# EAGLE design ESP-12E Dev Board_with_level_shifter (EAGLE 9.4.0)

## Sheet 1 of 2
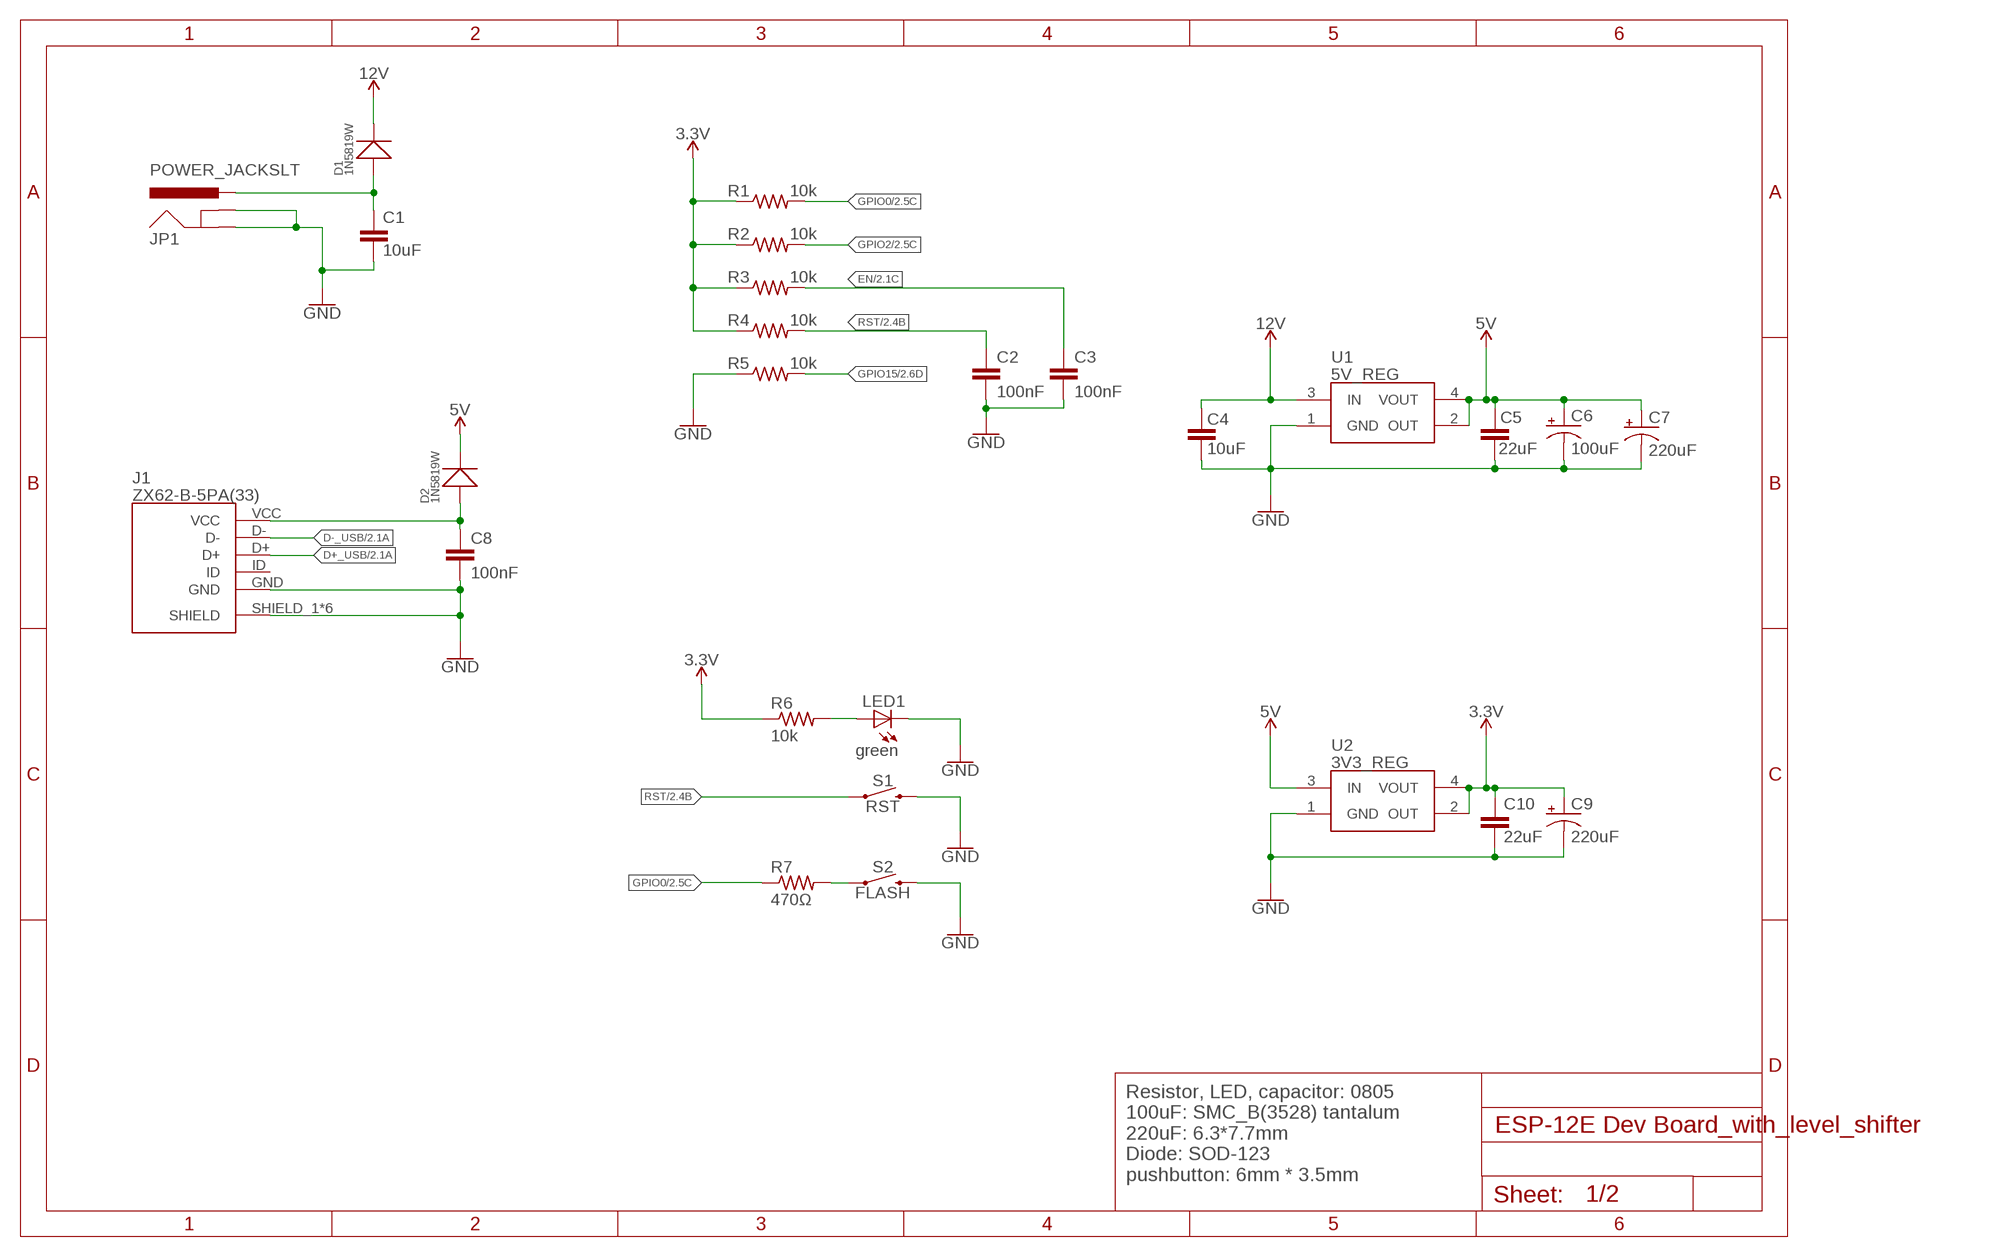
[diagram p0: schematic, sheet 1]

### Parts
C1  10uF  C-EUC0805  [C0805]
C2  100nF  C-EUC0805  [C0805]
C3  100nF  C-EUC0805  [C0805]
C4  10uF  C-EUC0805  [C0805]
C5  22uF  C-EUC0805  [C0805]
C6  100uF  CPOL-USSMCB  [SMC_B]
C7  220uF  CPOL-USUD-6,3X7,7  [UD-6,3X7,7_NICHICON]
C8  100nF  C-EUC0805  [C0805]
C9  220uF  CPOL-USUD-6,3X7,7  [UD-6,3X7,7_NICHICON]
C10  22uF  C-EUC0805  [C0805]
D1  1N5819W  SMD-DIODE-SCHOTTKY-20V-500MA(SOD-123)  [SOD-123]
D2  1N5819W  SMD-DIODE-SCHOTTKY-20V-500MA(SOD-123)  [SOD-123]
J1  ZX62-B-5PA(33)  [ZX62B5PA33]
JP1  POWER_JACKSLT  [POWER_JACK_SLOT]
LED1  green  LEDCHIP-LED0805  [CHIP-LED0805]
R1  10k  R-US_R0805  [R0805]
R2  10k  R-US_R0805  [R0805]
R3  10k  R-US_R0805  [R0805]
R4  10k  R-US_R0805  [R0805]
R5  10k  R-US_R0805  [R0805]
R6  10k  R-US_R0805  [R0805]
R7  470Ω  R-US_R0805  [R0805]
S1  RST  MOMENTARY-SWITCH-SPST-SMD-6.0X3.5MM  [TACTILE_SWITCH_SMD_6.0X3.5MM]
S2  FLASH  MOMENTARY-SWITCH-SPST-SMD-6.0X3.5MM  [TACTILE_SWITCH_SMD_6.0X3.5MM]
U1  5V_REG  AZ1117H-5.0TRE1  [SOT230P700X170-4N]
U2  3V3_REG  AZ1117H-5.0TRE1  [SOT230P700X170-4N]

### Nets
3.3V [power]: C9.+ C10.2 R1.1 R2.1 R3.1 R4.1 R6.1 U2.2(OUT) U2.4(VOUT) ; also sheet 2
5V [power]: C5.1 C6.+ C7.+ D2.- U1.2(OUT) U1.4(VOUT) U2.3(IN) ; also sheet 2
12V [power]: C4.1 D1.- U1.3(IN) ; also sheet 2
D+_USB: J1.D+ ; also sheet 2
D-_USB: J1.D- ; also sheet 2
EN: C3.2 R3.2 ; also sheet 2
GND [power]: C1.1 C2.1 C3.1 C4.2 C5.2 C6.- C7.- C8.1 C9.- C10.1 J1.GND J1.SHIELD_1(SHIELD) J1.SHIELD_2(SHIELD) J1.SHIELD_3(SHIELD) J1.SHIELD_4(SHIELD) J1.SHIELD_5(SHIELD) J1.SHIELD_6(SHIELD) JP1.GND@1(GNDBREAK) JP1.GND@2(GND) LED1.C R5.1 S1.2 S2.2 U1.1(GND) U2.1(GND) ; also sheet 2
GPIO0: R1.2 R7.1 ; also sheet 2
GPIO2: R2.2 ; also sheet 2
GPIO15: R5.2 ; also sheet 2
N$3: C1.2 D1.+ JP1.PWR
N$4: LED1.A R6.2
N$10 [power]: C8.2 D2.+ J1.VCC
POWER1: R7.2 S2.1
RST: C2.2 R4.2 S1.1 ; also sheet 2
Unconnected: J1.ID

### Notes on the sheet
- Resistor, LED, capacitor: 0805
  100uF: SMC_B(3528) tantalum
  220uF: 6.3*7.7mm
  Diode: SOD-123
  pushbutton: 6mm * 3.5mm

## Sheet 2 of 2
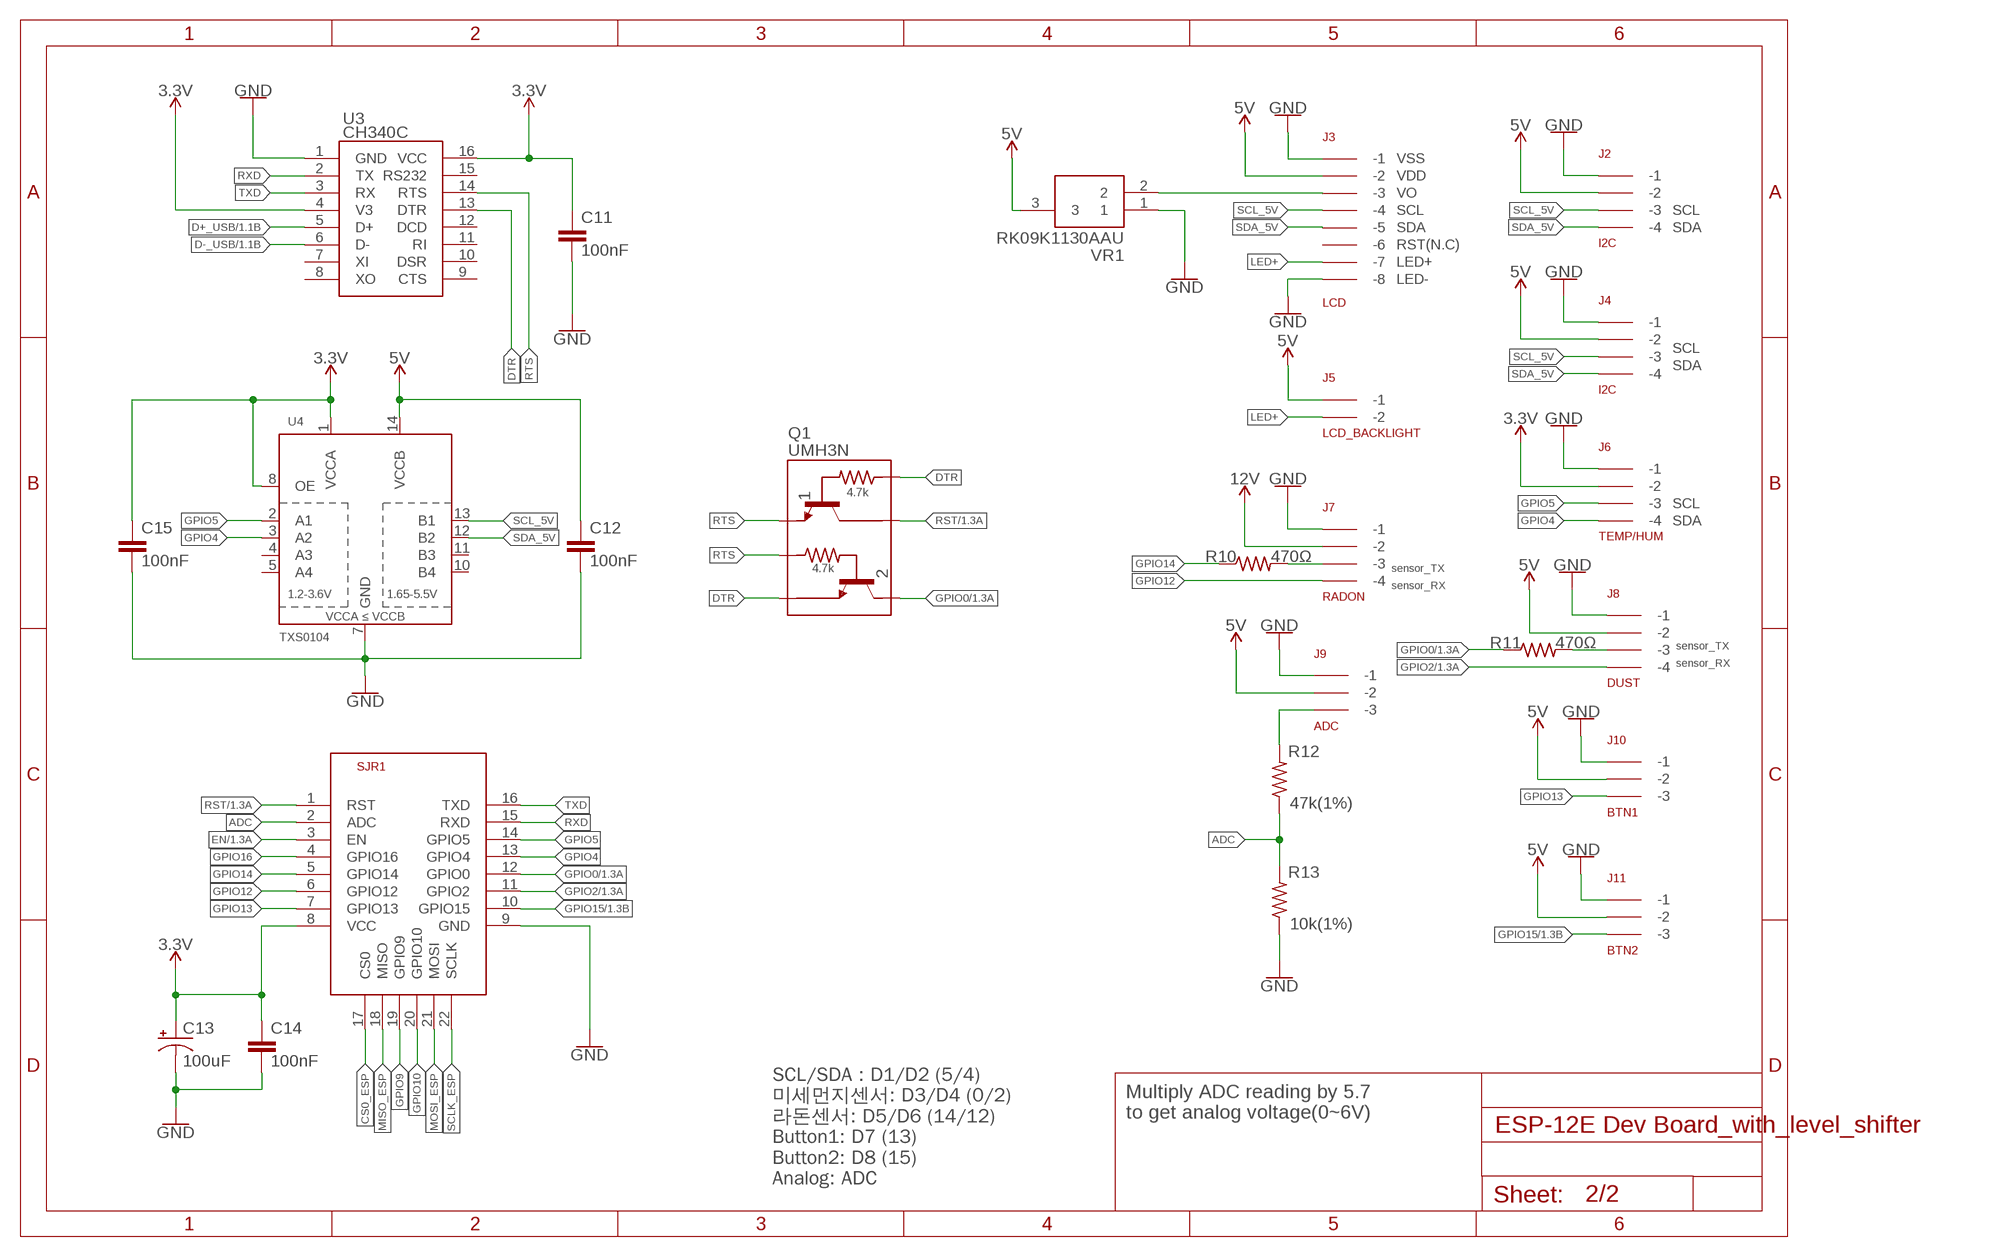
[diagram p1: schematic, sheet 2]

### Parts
C11  100nF  C-EUC0805  [C0805]
C12  100nF  C-EUC0805  [C0805]
C13  100uF  CPOL-USSMCB  [SMC_B]
C14  100nF  C-EUC0805  [C0805]
C15  100nF  C-EUC0805  [C0805]
J2  I2C  5267-4  [5267-4]
J3  LCD  5267-8  [5267-8]
J4  I2C  5267-4  [5267-4]
J5  LCD_BACKLIGHT  5267-2  [5267-2]
J6  TEMP/HUM  5267-4  [5267-4]
J7  RADON  5267-4  [5267-4]
J8  DUST  5267-4  [5267-4]
J9  ADC  5267-3  [5267-3]
J10  BTN1  5267-3  [5267-3]
J11  BTN2  5267-3  [5267-3]
Q1  UMH3N  UMH3NFHATN  [SOT65P210X100-6N]
R10  470Ω  R-US_R0805  [R0805]
R11  470Ω  R-US_R0805  [R0805]
R12  47k(1%)  R-US_R0805  [R0805]
R13  10k(1%)  R-US_R0805  [R0805]
SJR1  ESP-12E  ESP8266-12EESP12E  [ESP8266-ESP12E]
U3  CH340C  CH340G  [SOIC16]
U4  TXS0104  TXB0104PWR  [TSSOP14]
VR1  RK09K1130AAU  RK09K1130A6S  [RK09K1130BGM]

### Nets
3.3V [power]: C11.2 C13.+ C14.2 C15.2 J6.P$2(-2) SJR1.8(VCC) U3.4(V3) U3.16(VCC) U4.1(VCCA) U4.8(OE) ; also sheet 1
5V [power]: C12.2 J2.P$2(-2) J3.P$2(-2) J4.P$2(-2) J5.P$1(-1) J8.P$2(-2) J9.P$2(-2) J10.P$2(-2) J11.P$2(-2) U4.14(VCCB) VR1.3 ; also sheet 1
12V [power]: J7.P$2(-2) ; also sheet 1
ADC: R12.1 R13.2 SJR1.2(ADC)
CS0_ESP: SJR1.17(CS0)
D+_USB: U3.5(D+) ; also sheet 1
D-_USB: U3.6(D-) ; also sheet 1
DTR: Q1.2 Q1.4 U3.13(DTR)
EN: SJR1.3(EN) ; also sheet 1
GND [power]: C11.1 C12.1 C13.- C14.1 C15.1 J2.P$1(-1) J3.P$1(-1) J3.P$8(-8) J4.P$1(-1) J6.P$1(-1) J7.P$1(-1) J8.P$1(-1) J9.P$1(-1) J10.P$1(-1) J11.P$1(-1) R13.1 SJR1.9(GND) U3.1(GND) U4.7(GND) VR1.1 ; also sheet 1
GPIO0: Q1.3 R11.1 SJR1.12(GPIO0) ; also sheet 1
GPIO2: J8.P$4(-4) SJR1.11(GPIO2) ; also sheet 1
GPIO4: J6.P$4(-4) SJR1.13(GPIO4) U4.3(A2)
GPIO5: J6.P$3(-3) SJR1.14(GPIO5) U4.2(A1)
GPIO9: SJR1.19(GPIO9)
GPIO10: SJR1.20(GPIO10)
GPIO12: J7.P$4(-4) SJR1.6(GPIO12)
GPIO13: J10.P$3(-3) SJR1.7(GPIO13)
GPIO14: R10.1 SJR1.5(GPIO14)
GPIO15: J11.P$3(-3) SJR1.10(GPIO15) ; also sheet 1
GPIO16: SJR1.4(GPIO16)
LED+: J3.P$7(-7) J5.P$2(-2)
MISO_ESP: SJR1.18(MISO)
MOSI_ESP: SJR1.21(MOSI)
N$2: J3.P$3(-3) VR1.2
N$5: J9.P$3(-3) R12.2
N$6: J7.P$3(-3) R10.2
N$9: J8.P$3(-3) R11.2
RST: Q1.6 SJR1.1(RST) ; also sheet 1
RTS: Q1.1 Q1.5 U3.14(RTS)
RXD: SJR1.15(RXD) U3.2(TX)
SCL_5V: J2.P$3(-3) J3.P$4(-4) J4.P$3(-3) U4.13(B1)
SCLK_ESP: SJR1.22(SCLK)
SDA_5V: J2.P$4(-4) J3.P$5(-5) J4.P$4(-4) U4.12(B2)
TXD: SJR1.16(TXD) U3.3(RX)
Unconnected: J3.P$6(-6) U3.7(XI) U3.8(XO) U3.9(CTS) U3.10(DSR) U3.11(RI) U3.12(DCD) U3.15(RS232) U4.4(A3) U4.5(A4) U4.10(B4) U4.11(B3)

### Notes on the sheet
- VSS
- VDD
- VO
- SCL | SCL
- SDA | SDA
- RST(N.C)
- LED+
- LED-
- SCL
- SDA
- SCL
- SDA
- sensor_TX
- sensor_RX
- sensor_TX
- sensor_RX
- SCL/SDA : D1/D2 (5/4)
  미세먼지센서: D3/D4 (0/2)
  라돈센서: D5/D6 (14/12)
  Button1: D7 (13)
  Button2: D8 (15)
  Analog: ADC
- Multiply ADC reading by 5.7
  to get analog voltage(0~6V)

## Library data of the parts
C1-C5 C8 C10-C12 C14 C15 = rcl:C-EU: CAPACITOR, European symbol; SPICEPREFIX: C
C6 C7 C9 C13 = rcl:CPOL-US: POLARIZED CAPACITOR, American symbol; SPICEPREFIX: C
D1 D2 = Seeed-Diode:SMD-DIODE-SCHOTTKY-20V-500MA(SOD-123): 304020032; MPN: SS0520-7-F; VALUE: 20V-500MA
J1 = SamacSys_Parts:ZX62-B-5PA(33): USB Connectors MICRO B RECEPT RA SMT BTTM MNT Source: Datasheet; DESCRIPTION: USB Connectors MICRO B RECEPT RA SMT BTTM MNT; HEIGHT: 2.8mm; MANUFACTURER_NAME: Hirose; MANUFACTURER_PART_NUMBER: ZX62-B-5PA(33); MOUSER_PART_NUMBER: 798-ZX62-B-5PA33; MOUSER_PRICE-STOCK: https://www.mouser.com/Search/Refine.aspx?Keyword=798-ZX62-B-5PA33
J2 J4 J6-J8 = con-molex-spox:5267-4
J3 = con-molex-spox:5267-8
J5 = con-molex-spox:5267-2
J9-J11 = con-molex-spox:5267-3
JP1 = kanflo:POWER_JACK: Power Jack This is the standard 5.5mm barrel jack for power. The SLT footprint has been proven in designs produced by DirtyPCBs.com and only works if the mill layer is transmitted to the PCB fab house and the fab house accepts it. Rumours has it OSH Park accepts this design too. This symbol is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
LED1 = adafruit:LED: LED
Q1 = SamacSys_Parts:UMH3NFHATN: ROHM - UMH3NFHATN - TRANS, NPN, AUTO, 4.7K/4.7K, SOT-353 Source: Datasheet; DESCRIPTION: ROHM - UMH3NFHATN - TRANS, NPN, AUTO, 4.7K/4.7K, SOT-353; HEIGHT: 1mm; MANUFACTURER_NAME: ROHM Semiconductor; MANUFACTURER_PART_NUMBER: UMH3NFHATN; MOUSER_PART_NUMBER: 755-UMH3NFHATN; MOUSER_PRICE-STOCK: https://www.mouser.com/Search/Refine.aspx?Keyword=755-UMH3NFHATN
R1-R7 R10-R13 = rcl:R-US_: RESISTOR, American symbol; SPICEPREFIX: R
S1 S2 = SparkFun-Switches:MOMENTARY-SWITCH-SPST: Momentary Switch (Pushbutton) - SPST; PROD_ID: SWCH-00815; SF_SKU: COM-08229
SJR1 = esp12e:ESP8266-12E: ESP8266-12E Library for Eagle CAD The author not responsible for any damages or errors!. Created by Suhail jr.lt;/author>
U1 U2 = SamacSys_Parts:AZ1117H-5.0TRE1: 1A 5V LDO Linear Voltage Reg SOT-223 Diodes Inc AZ1117H-5.0TRE1, Single Linear Voltage Regulator, 1A 4.9 5.1 V, 1%, 3-Pin SOT-223 Source: Datasheet; DESCRIPTION: 1A 5V LDO Linear Voltage Reg SOT-223 Diodes Inc AZ1117H-5.0TRE1, Single Linear Voltage Regulator, 1A 4.9 5.1 V, 1%, 3-Pin SOT-223; HEIGHT: 1.7mm; MANUFACTURER_NAME: Diodes Inc.; MANUFACTURER_PART_NUMBER: AZ1117H-5.0TRE1; MOUSER_PART_NUMBER: 621-AZ1117H-5.0TRE1; MOUSER_PRICE-STOCK: https://www.mouser.com/Search/Refine.aspx?Keyword=621-AZ1117H-5.0TRE1
U3 = ch340g:CH340G
U4 = SparkFun-IC-Comms:TXB0104PWR: 4-Bit Bi-Directional Level Shifter 1.2V-3.6V (VCCA) to 1.65V-5.5V (VCCB) bi-directional level shifter with auto direction sensing. Max data rate - VCCA 1.8V: 20Mbps (50ns), VCCA 3.3V: 100Mbps (10ns) Digikey: 296-21929-1-ND (TSSOP) Datasheet SparkFun Products SparkFun Cellular Shield - MG2639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; PROD_ID: NA-XXXXX; VALUE: TXB0104
VR1 = SamacSys_Parts:RK09K1130A6S: Audio single pot. 10K Vertical 15mm,1B Alps RK09K Series, Linear Potentiometer with a 6 mm Dia. Shaft, 10k, +/-20%, Through Hole Source: Datasheet; DESCRIPTION: Audio single pot. 10K Vertical 15mm,1B Alps RK09K Series, Linear Potentiometer with a 6 mm Dia. Shaft, 10k, +/-20%, Through Hole; HEIGHT: mm; MANUFACTURER_NAME: ALPS; MANUFACTURER_PART_NUMBER: RK09K1130A6S; MOUSER_PART_NUMBER: 688-RK09K1130A6S; MOUSER_PRICE-STOCK: https://www.mouser.com/Search/Refine.aspx?Keyword=688-RK09K1130A6S

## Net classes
1 power: width 0.457 mm

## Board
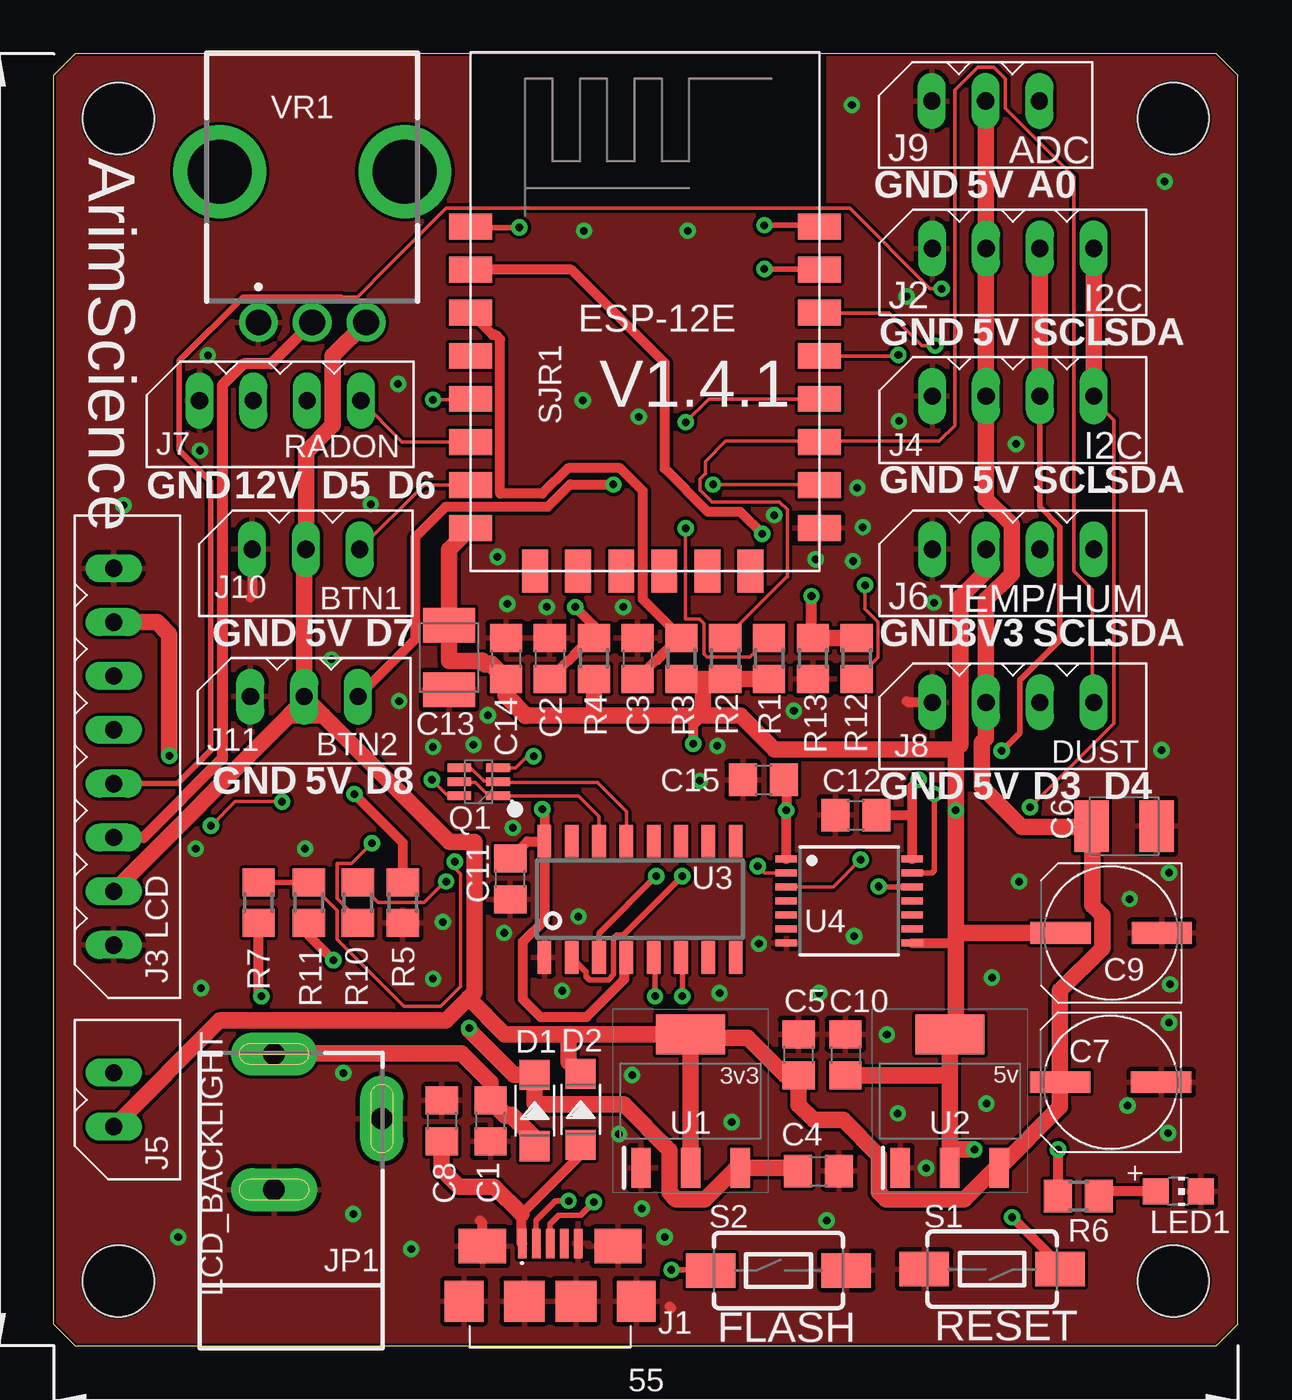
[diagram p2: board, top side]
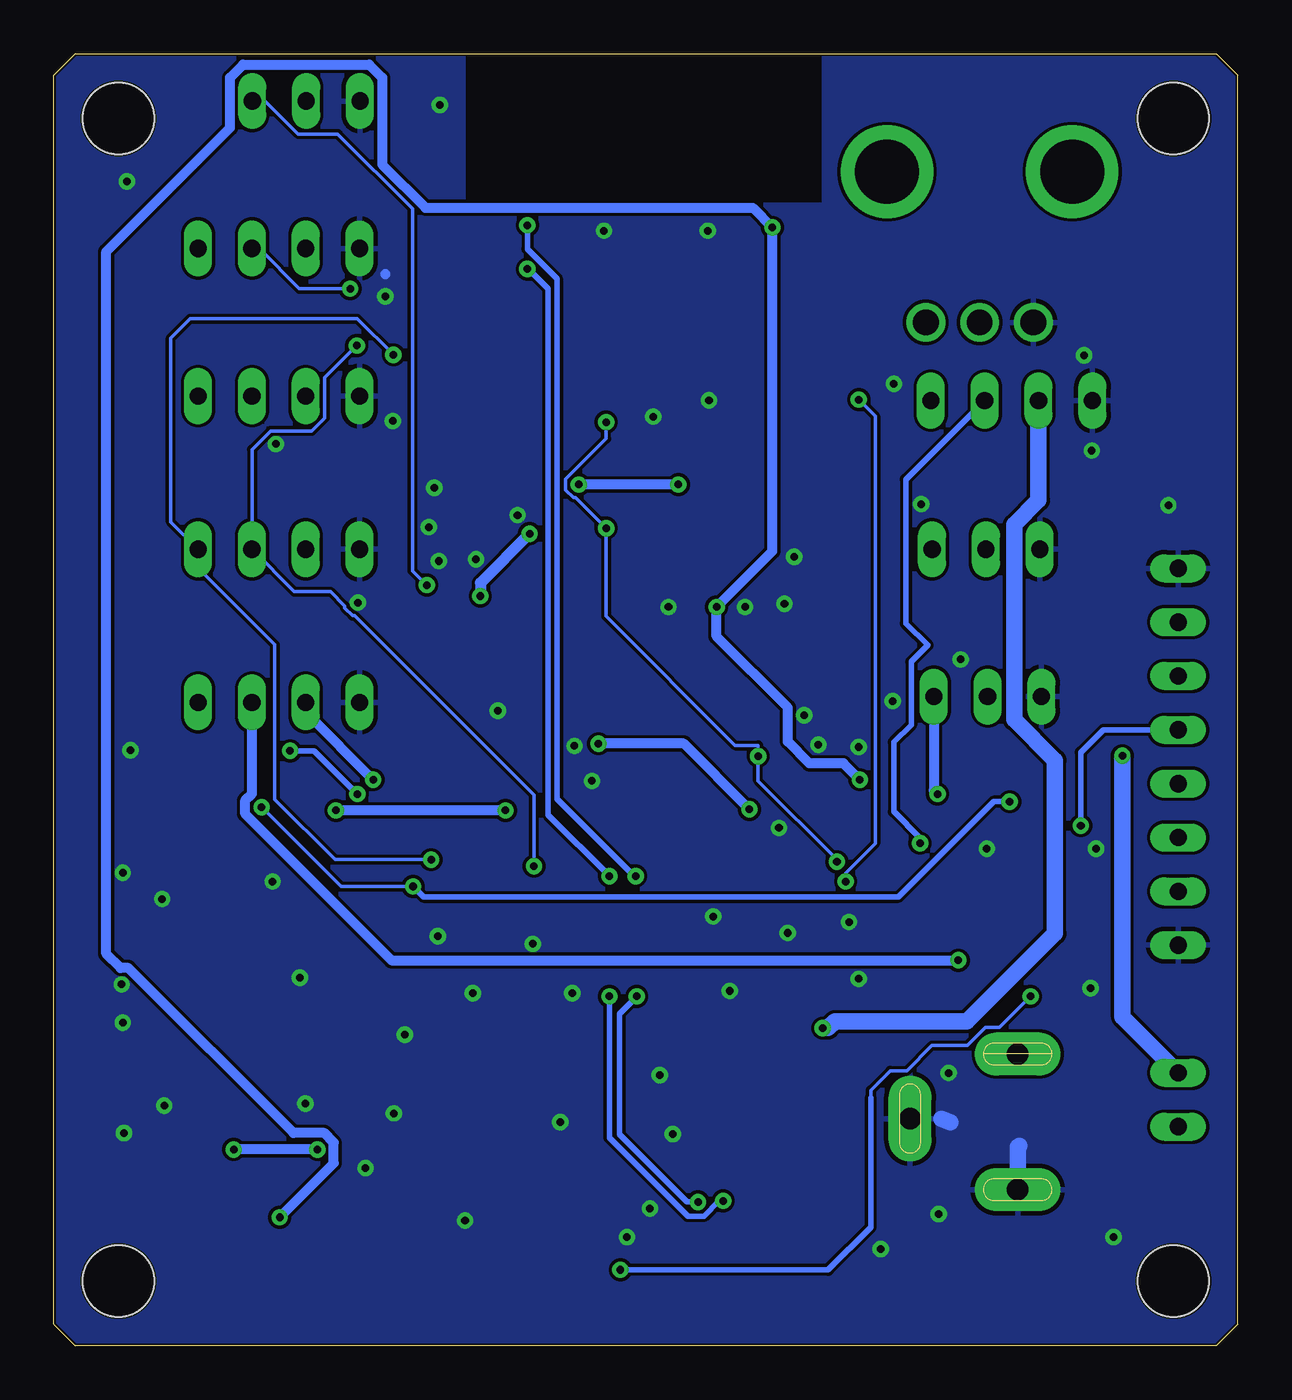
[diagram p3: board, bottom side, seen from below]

Size 55 x 60 mm. Coordinates in mm from the lower left corner, seen from the top.
Outline: 0,1 0,59 1,60 54,60 55,59 55,1 54,0 1,0 0,1
Copper layers (1*16): Top 0.035mm / dielectric 1.5mm / Bottom 0.035mm
Design rules "default *": minimum track width 6mil, minimum drill 0.35mm, track to track 6mil, track to pad 6mil, pad to pad 6mil, via to via 6mil, smd to smd 6mil, copper to edge 4mil, drill to drill 6mil, minimum pad ring 10mil, minimum via ring 8mil, stop-mask expansion 4mil, vias tented up to drill 15mil, thermal gap 8mil
Holes 3.3 mm at 3,57 52,57 52,3 3,3

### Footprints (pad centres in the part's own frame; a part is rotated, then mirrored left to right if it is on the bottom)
C0805 = smd 1.3 x 1.5: 1 -0.95,0; 2 0.95,0
SMC_B = smd 1.6 x 2.4: + -1.5,0; - 1.5,0
UD-6,3X7,7_NICHICON = smd 2.8 x 1: + 2.35,0; - -2.35,0
SOD-123 = smd 1.397 x 1.397: + -1.651,0; - 1.651,0
ZX62B5PA33 = smd 0.4 x 1.35: D+ 0,1.95; D- -0.65,1.95; GND 1.3,1.95; ID 0.65,1.95; VCC -1.3,1.95 | smd 2.2 x 1.6: SHIELD_1 -3.15,1.825; SHIELD_6 3.15,1.825 | smd 1.8 x 1.9: SHIELD_2 -4,-0.725; SHIELD_5 4,-0.725 | smd 1.9 x 1.9: SHIELD_3 -1.2,-0.725; SHIELD_4 1.2,-0.725
5267-4 = drill 0.8 long: P$1 0,0; P$2 2.5,0; P$3 5,0; P$4 7.5,0
5267-8 = drill 0.8 long: P$1 0,0; P$2 2.5,0; P$3 5,0; P$4 7.5,0; P$5 10,0; P$6 12.5,0; P$7 15,0; P$8 17.5,0
5267-2 = drill 0.8 long: P$1 0,0; P$2 2.5,0
5267-3 = drill 0.8 long: P$1 0,0; P$2 2.5,0; P$3 5,0
POWER_JACK_SLOT = drill 1 pad 2 long: GND@1 2.5,1.39; GND@2 -2.5,-1.91; PWR 2.5,-4.91
CHIP-LED0805 = smd 1.2 x 1.2: A 0,-1.05; C 0,1.05
SOT65P210X100-6N = smd 1.1 x 0.4: 1 -0.9,0.65; 2 -0.9,0; 3 -0.9,-0.65; 4 0.9,-0.65; 5 0.9,0; 6 0.9,0.65
R0805 = smd 1.3 x 1.5: 1 -0.95,0; 2 0.95,0
TACTILE_SWITCH_SMD_6.0X3.5MM = smd 2.3 x 1.6: 1 -3.15,0; 2 3.15,0
ESP8266-ESP12E = smd 2 x 1.2: 1 -7.62,5.84; 2 -7.62,3.84; 3 -7.62,1.84; 4 -7.62,-0.16; 5 -7.62,-2.16; 6 -7.62,-4.16; 7 -7.62,-6.16; 8 -7.62,-8.16; 9 8.58,-8.16; 10 8.58,-6.16; 11 8.58,-4.16; 12 8.58,-2.16; 13 8.58,-0.16; 14 8.58,1.84; 15 8.58,3.84; 16 8.58,5.84 | smd 1.2 x 2: 17 -4.62,-10.16; 18 -2.62,-10.16; 19 -0.62,-10.16; 20 1.38,-10.16; 21 3.38,-10.16; 22 5.38,-10.16
SOT230P700X170-4N = smd 1.85 x 0.9: 1 -3.1,2.3; 2 -3.1,0; 3 -3.1,-2.3 | smd 1.85 x 3.2: 4 3.1,0
SOIC16 = smd 0.635 x 1.524: 1 -4.445,-2.695; 2 -3.175,-2.695; 3 -1.905,-2.695; 4 -0.635,-2.695; 5 0.635,-2.695; 6 1.905,-2.695; 7 3.175,-2.695; 8 4.445,-2.695; 9 4.445,2.695; 10 3.175,2.695; 11 1.905,2.695; 12 0.635,2.695; 13 -0.635,2.695; 14 -1.905,2.695; 15 -3.175,2.695; 16 -4.445,2.695
TSSOP14 = smd 0.305 x 0.991: 1 -1.95,-2.918; 2 -1.3,-2.918; 3 -0.65,-2.918; 4 0,-2.918; 5 0.65,-2.918; 6 1.3,-2.918; 7 1.95,-2.918; 8 1.95,2.918; 9 1.3,2.918; 10 0.65,2.918; 11 0,2.918; 12 -0.65,2.918; 13 -1.3,2.918; 14 -1.95,2.918
RK09K1130BGM = drill 1.2 pad 1.8: 1 -2.5,-12.5; 2 0,-12.5; 3 2.5,-12.5 | drill 2.97 pad 4.3: 4 4.3,-5.5; 5 -4.3,-5.5

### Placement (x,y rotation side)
C1  20.29,10.43 90 top
C2  23.03,31.92 270 top
C3  27.11,31.92 270 top
C4  35.52,8.11 0 top
C5  34.59,13.51 90 top
C6  49.71,24.13 0 top
C7  49.08,12.23 180 top
C8  18.02,10.43 270 top
C9  49.11,19.17 180 top
C10  36.77,13.51 270 top
C11  21.2,21.68 90 top
C12  37.24,24.64 0 top
C13  18.36,31.96 270 top
C14  21,31.91 270 top
C15  32.95,26.28 0 top
D1  22.34,10.92 90 top
D2  24.47,10.97 90 top
J1  23.05,2.79 0 top
J2  40.8,50.96 0 top
J3  2.78,18.6 90 top
J4  40.8,44.1 0 top
J5  2.78,10.17 90 top
J6  40.8,36.99 0 top
J7  6.76,43.9 0 top
J8  40.8,29.88 0 top
J9  40.78,57.81 0 top
J10  9.21,36.99 0 top
J11  9.13,30.15 0 top
JP1  12.73,8.64 180 top
LED1  52.23,7.16 270 top
Q1  19.73,26.19 180 top
R1  33.22,31.92 90 top
R2  31.19,31.92 90 top
R3  29.15,31.92 90 top
R4  25.09,31.92 90 top
R5  16.21,20.57 90 top
R6  47.59,6.95 0 top
R7  9.51,20.57 270 top
R10  14.13,20.57 270 top
R11  11.84,20.57 270 top
R12  37.29,31.92 270 top
R13  35.26,31.92 90 top
S1  43.58,3.56 180 top
S2  33.65,3.49 0 top
SJR1  26.97,46.13 0 top
U1  29.57,11.37 90 top
U2  41.61,11.37 90 top
U3  27.23,20.73 0 top
U4  36.94,20.66 270 top
VR1  12,60.02 0 top

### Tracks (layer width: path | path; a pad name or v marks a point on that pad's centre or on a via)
3.3V  (via drill 0.35)
  Top 0.457: U4.1 v34.02,24.86 | v34.02,24.86 | U4.8 41.85,18.7 41.89,18.66 | v29.7,27.96 29.7,28.82 30.16,29.28 | C11.2 22,23.43 U3.16 | v22.69,24.91 22.78,24.82 U3.16 | U3.4 26.5,17.95 26.5,17.03 24.75,15.27 22.61,15.27 21.78,16.1 21.78,18.76 22.78,19.76 U3.16 | C15.2 34.02,26.16 v34.02,24.86 | v46.64,9.11 R6.1
  Top 0.762: R3.1 30.16,30.97 | 30.16,30.97 R2.1 R1.1 | J6.P$2 43.3,35.95 42.11,34.76 42.11,27.91 41.89,27.69 | v42.76,9.11 41.61,9.11 U2.2 41.61,12.62 | 41.89,27.69 v41.89,24.86 41.89,19.17 | SJR1.8 18.36,36.98 C13.+ 18.36,31.8 18.37,31.79 19.86,31.79 | 30.16,29.28 31.89,29.28 33.48,27.69 41.89,27.69 | 30.16,30.97 30.16,29.28 | 41.89,19.17 41.89,18.66 41.89,14.75 U2.4 41.61,12.62 | C9.+ 41.89,19.17 | C10.2 41.56,12.56 41.61,12.62 | 30.16,29.28 25.08,29.28 | 25.08,29.28 21.92,29.28 | 25.08,29.28 R4.1
  Top 0.813: 21.92,29.28 21,30.2 C14.2 20.31,31.65 20.02,31.65 19.88,31.79 19.86,31.79
  Bottom 0.457: v34.02,24.86 v41.89,24.86 | v22.69,24.91 25.74,27.96 v29.7,27.96 | v42.76,9.11 v46.64,9.11
5V  (via drill 0.35)
  Top 0.457: 39.86,24.66 39.86,25.98 v40.17,26.28 | 39.86,24.66 39.86,22.65 U4.14 | C12.2 38.21,24.66 39.86,24.66
  Top 0.762: J9.P$2 43.28,50.98 J2.P$2 J4.P$2 43.3,39.32 44.49,38.14 44.49,35.84 43.3,34.66 J8.P$2 43.3,28.19 43.12,28.01 43.12,25.96 44.97,24.1 48.18,24.1 C6.+ 48.24,24.09 48.24,20.44 48.69,19.99 48.69,18.45 46.73,16.49 C7.+ 46.73,11.09 U2.3 43.74,8.27 42.28,6.81 38.64,6.81 38.33,7.12 38.33,8.82 36.67,10.48 35.3,10.48 34.59,11.2 C5.1 33.98,12.56 32.24,14.3 29.74,14.3 U1.4 | J11.P$2 11.63,36.91 J10.P$2 11.71,41.51 12.95,42.75 12.95,45.98 VR1.3 | J3.P$2 10.94,29.26 | 10.94,29.26 11.63,29.95 J11.P$2 | J11.P$2 12.51,29.26 | 12.51,29.26 18.38,23.4 19.54,23.4 19.54,16.42 19.27,16.14 | 12.51,29.26 10.94,29.26 | 19.27,16.14 18.23,15.11 7.71,15.11 J5.P$1 | 19.27,16.14 20.94,14.47 23.91,14.47 | U1.4 23.91,14.47 | U1.2 U1.4 | D2.- 23.91,13.18 23.91,14.47
  Bottom 0.457: v40.17,26.28 43.29,29.41 43.29,29.81 J8.P$2
12V  (via drill 0.35)
  Top 0.762: v19.29,14.75 19.29,14.66 21.37,12.57 D1.- 22.34,11.25 22.38,11.2 26.47,11.2 28.59,9.08 28.59,7.12 28.9,6.81 30.25,6.81 31.7,8.27 U1.3 34.42,8.27 C4.1
  Bottom 0.762: v19.29,14.75 19.03,14.75 18.73,15.06 12.58,15.06 8.5,19.14 8.5,27.19 10.39,29.08 10.39,38.14 9.26,39.27 J7.P$2
ADC  (via drill 0.35)
  Top 0.457: v32.9,37.71 31.89,38.73 30.38,38.73 28.38,40.73 28.38,45.64 24.04,49.97 SJR1.2
  Top 0.508: R13.2 35.19,32.94 v35.19,34.82
  Top 0.762: R12.1 R13.2
  Bottom 0.508: v32.9,37.71 35.19,35.43 v35.19,34.82
D+_USB  (via drill 0.35)
  Top 0.254: v27.92,16.22 27.92,17.98 U3.5 | v25.08,6.67 24.47,6.06 23.45,6.06 23.05,5.67 J1.D+
  Bottom 0.254: v25.08,6.67 25.59,6.67 28.74,9.82 28.74,15.41 v27.92,16.22
D-_USB  (via drill 0.35)
  Top 0.254: v29.19,16.22 29.19,17.98 U3.6 | v23.91,6.72 23.3,6.72 22.4,5.83 J1.D-
  Bottom 0.254: v29.19,16.22 29.19,9.66 25.55,6.02 24.81,6.02 24.1,6.72 v23.91,6.72
DTR
  Top 0.152: Q1.4 18.91,26.84 19.36,26.84 19.97,26.23 20.58,26.23 Q1.2 20.66,26.16 25.26,26.16 26.59,24.82 U3.13
EN
  Top 0.457: SJR1.3 20.37,46.95 20.51,46.95 20.73,46.73 20.73,39.56 22.68,39.56 23.88,40.76 26.31,40.76 27.36,39.7 27.36,34.66 R3.2 29.01,32.87 28.24,32.1 28.24,32.06 28.02,31.84 27.98,31.84 C3.2
GND  (via drill 0.35)
  Top 0.457: J8.P$1 39.67,29.88 39.61,29.94 | J1.SHIELD_2 18.98,2 | 28.62,1.81 28.69,1.75 | J1.SHIELD_1 19.9,5.7 19.8,5.81 | J10.P$1 9.21,34.85 9.13,34.77
  Bottom 0.457: 39.61,49.77 39.61,49.75
  Bottom 0.762: JP1.GND@1 10.23,9.23 10.14,9.28 | 13.77,10.55 13.36,10.38
  other vias: 16.6,4.49 24.62,51.78 29.45,51.78 24.57,43.91 27.16,43.15 30.01,26.23 30.92,16.38 6.59,23.08 11.67,23.08 5.78,5.05 15.99,44.67 14.72,39.08 43.57,17.09 51.85,16.78 44.84,21.56 51.75,9.87 26.86,12.57 31.48,10.38 27.31,6.37 37.58,38.02 40.88,34.51 6.79,41.57 34.38,29.48 20.15,29.28 19.49,27.91 30.82,27.86 13.9,6.11 17.61,17.04 3.24,39.03 6.84,16.61 37.07,57.63 44.69,41.88 51.8,15 51.8,21.96 43.32,11.25 40.52,8.25 33.46,38.58 13.45,12.67 39.61,48.74 39.25,42.94 7.15,45.99 23.61,16.48 26.25,9.82 35.9,5.81 37.12,36.44 20.61,36.65 21.07,34.46 24.37,19.93 49.97,20.75 49.87,11.14 39.2,10.79 35.54,16.38 22.89,34.31 17.61,27.81 35.39,36.52 37.32,39.85 51.6,54.07 12.89,31.87 18.07,19.68 28.38,5.05 51.44,27.65 26.45,34.31 16.04,29.94 38.69,14.45 37.17,19.02 32.75,18.66 21.32,24.05 20.91,19.17
  pour Top: -6.89,65.66 -6.89,-4.32 57.72,-4.32 57.72,65.66
  pour Bottom: -6.86,65.66 -6.86,-4.35 58.72,-4.35 58.72,65.66
GPIO0  (via drill 0.35)
  Top 0.152: v22.29,27.38 21.98,27.38 21.45,26.84 Q1.3 | v18.63,22.47 18.63,22.17 18.88,21.91 18.88,16.68 17.97,15.77 16.26,15.77 13.15,18.88 13.15,20.22 R11.1 | v29.35,42.89 30.43,43.97 SJR1.12 | R1.2 32.34,31.99 30.34,31.99 30.21,32.13 30.21,33.54 30,33.75 29.35,33.75 v29.35,37.97
  Top 0.254: R7.1 R11.1
  Bottom 0.152: v18.63,22.47 18.63,22.57 22.29,26.23 v22.29,27.38 22.29,27.88 23.35,27.88 29.35,33.88 v29.35,37.97 30.77,39.39 30.87,39.39 31.22,39.75 31.22,40.25 29.35,42.13 v29.35,42.89
GPIO2
  Top 0.152: SJR1.11 35.59,42.01 | J8.P$4 48.24,29.89 48.24,35.12 47.38,35.98 47.38,54.3 44.2,57.47 44.2,58.84 43.67,59.38 42.91,59.38 41.84,58.31 41.84,42.74 41.11,42.01 35.59,42.01 | 35.59,42.01 31.2,42.01 30.26,41.06 30.26,40.5 30.01,40.25 30.01,39.75 30.57,39.18 33.71,39.18 34.07,38.83 34.07,35.7 34.02,35.7 R2.2
GPIO4  (via drill 0.35)
  Top 0.152: v39.23,46.02 39.18,45.97 35.59,45.97 SJR1.13 | U4.3 36.2,21.3 v37.47,22.57
  Bottom 0.152: v39.23,46.02 40.9,47.7 48.68,47.7 49.56,46.81 49.56,38.26 J6.P$4 48.24,36.98 48.24,36.06 44.74,32.56 44.74,25.37 41.95,22.57 v37.47,22.57
GPIO5  (via drill 0.35)
  Top 0.152: v40.93,46.45 40.32,46.45 38.82,47.95 35.59,47.95 SJR1.14 | U4.2 33.01,21.95 v32.7,22.27
  Bottom 0.152: v40.93,46.45 42.42,44.96 42.42,43.08 43.02,42.48 44.94,42.48 45.8,41.62 J6.P$3 43.83,35.02 42.15,35.02 41.48,34.36 41.48,34.26 41.13,33.91 41.03,33.91 32.7,25.57 32.7,25.46 32.7,25.42 v32.7,22.27
GPIO12
  Top 0.152: J7.P$4 16.19,41.97 SJR1.6
GPIO13
  Top 0.152: J10.P$3 17.19,39.97 SJR1.7
GPIO14  (via drill 0.35)
  Top 0.152: v18.22,21.56 18.17,21.56 17.2,20.59 15.06,20.59 R10.1 | v17.61,43.94 19.31,43.94 SJR1.5
  Bottom 0.152: v18.22,21.56 18.22,21.96 16.85,23.34 16.85,43.17 v17.61,43.94
GPIO15  (via drill 0.35)
  Top 0.152: v30.62,40 35.53,40 SJR1.10
  Top 0.457: v25.99,40 23.98,40 22.94,38.95 18.19,38.95 16.78,37.54 16.78,32.8 J11.P$3 | v13.95,25.62 16.21,23.37 R5.2
  Bottom 0.457: v25.99,40 v30.62,40 | J11.P$3 14.13,25.8 v13.95,25.62
LED+  (via drill 0.35)
  Top 0.762: v5.37,27.4 5.37,33.04 4.8,33.6 J3.P$7
  Bottom 0.762: J5.P$2 5.37,15.27 v5.37,27.4
N$2
  Top 0.508: VR1.2 10.09,45.61 8.82,45.61 7.82,44.61 7.82,27.26 4.16,23.6 J3.P$3
N$3
  Top 0.762: C1.2 20.29,12.23 18.93,13.58 10.27,13.58 JP1.PWR
  Top 0.813: C1.2 20.98,10.69 21.27,10.69 22.34,9.62 D1.+
N$4
  Top 0.457: LED1.A 48.75,7.16 R6.2
N$5  (via drill 0.35)
  Top 0.152: v37.68,35.33 37.68,34.21 38.27,33.62 38.27,31.95 R12.2
  Bottom 0.152: v37.68,35.33 38.34,35.98 38.34,52.8 41.81,56.27 43.65,56.27 45.18,57.81 J9.P$3
N$6  (via drill 0.35)
  Top 0.152: R10.2 14.13,19.8 13.15,20.78 13.15,22.4 13.83,22.4 v14.77,23.34
  Bottom 0.254: J7.P$3 15.43,40.23 15.43,33.55 14.41,32.53 15.17,31.77 15.17,28.84 15.98,28.03 15.98,24.81 14.77,23.59 v14.77,23.34
N$9  (via drill 0.35)
  Top 0.457: v12.99,17.9 11.84,19.05 R11.2
  Bottom 0.457: J8.P$3 45.8,25.63 46.11,25.33 46.11,24.7 39.31,17.9 v12.99,17.9
N$10
  Top 0.457: J1.VCC 21.72,4.78 21.72,6.11 24.47,8.87 D2.+
  Top 0.762: 21.72,6.11 20.45,7.38 18.83,7.38 18.02,8.2 C8.2
POWER1  (via drill 0.35)
  Top 0.254: v28.69,3.52 30.47,3.52 S2.1
  Top 0.457: v9.64,16.22 9.51,16.35 R7.2
  Bottom 0.152: 17.05,11.5 17.05,11.87 16.15,12.78 15.37,12.78 14.21,13.94 12.58,13.94 11.74,14.78 11.09,14.78 v9.64,16.22
  Bottom 0.254: 17.05,11.5 17.05,5.5 19.03,3.52 v28.69,3.52
RST  (via drill 0.35)
  Top 0.152: v17.56,26.28 18.3,25.54 Q1.6
  Top 0.254: v21.62,51.94 19.39,51.94 SJR1.1
  Top 0.457: C2.2 23.9,31.84 23.94,31.84 24.17,32.06 24.17,32.1 24.94,32.87 R4.2 25.09,33.43 v24.22,34.31 | v44.51,5.96 46.73,3.75 S1.1
  Bottom 0.457: v44.51,5.96 42,8.48 42,9.43 42.44,9.87 43.87,9.87 51.54,17.54 51.9,17.54 52.56,18.2 52.56,50.82 46.81,56.57 46.81,58.89 46.21,59.5 40.35,59.5 39.74,58.89 39.74,54.85 37.74,52.85 22.54,52.85 v21.62,51.94 21.62,36.9 v24.22,34.31 24.22,32.94 20.91,29.63 20.91,28.05 19.91,27.05 18.33,27.05 v17.56,26.28
RTS
  Top 0.152: Q1.5 18.91,26.16 19.59,26.16 20.2,25.55 20.58,25.55 Q1.1 24.37,25.54 25.32,24.59 U3.14
RXD  (via drill 0.35)
  Top 0.254: v33,50.01 35.52,50.01 SJR1.15 | v29.19,21.81 26.46,19.08 26.16,19.08 25.99,18.92 25.99,17.24 25.75,17 24.89,17 24.72,17.16 24.72,17.37 U3.2
  Bottom 0.152: 32.95,50.01 v33,50.01
  Bottom 0.254: 32.95,50.01 32.04,49.09 32.04,24.66 v29.19,21.81
SCL_5V  (via drill 0.35)
  Top 0.152: 3.03,26.1 J3.P$4 | v41.23,49.09 40.7,49.09 36.97,52.83 18.22,52.83 15.53,50.13 14.11,48.71 13.34,48.71
  Top 0.254: v44.03,27.63 44.87,28.47 44.87,30.92 46.73,32.78 46.73,38.03 45.8,38.96 J4.P$3 | 3.03,26.1 5.75,26.1 7.29,27.65 7.29,40.14 5.83,41.6 5.83,45.74 8.8,48.71 13.34,48.71 | U4.13 40.78,21.95 40.9,22.08 v40.9,25.62
  Top 0.762: J2.P$3 J4.P$3
  Bottom 0.152: v41.23,49.09 43.6,49.09 45.42,50.92 45.73,50.92 J2.P$3
  Bottom 0.254: v40.9,25.62 42.91,27.63 v44.03,27.63
SDA_5V  (via drill 0.35)
  Top 0.152: v45.35,25.01 49.23,28.9 49.23,43 48.47,43.76 J4.P$4 | v7.3,24.15 8.42,25.27 v10.6,25.27
  Top 0.254: U4.12 38.34,21.3 v38.31,21.33
  Top 0.762: J4.P$4 J2.P$4
  Bottom 0.152: v45.35,25.01 41.66,21.33 v38.31,21.33
  Bottom 0.254: v38.31,21.33 37.83,20.85 15.76,20.85 11.35,25.27 v10.6,25.27 | J3.P$5 6.25,28.6 7.3,27.55 v7.3,24.15
TXD  (via drill 0.35)
  Top 0.254: v33,52.04 35.49,52.04 SJR1.16 | U3.3 25.32,19.16 v27.98,21.81
  Bottom 0.254: v33,52.04 33,50.94 31.63,49.56 31.63,25.4 28.04,21.81 v27.98,21.81

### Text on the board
tPlace: ArimScience | GND | 5V | A0 | GND | 5V | SCL | SDA | V1.4.1 | GND | 5V | SCL | SDA | GND | 12V | D5 | D6 | GND | 5V | D7 | GND | 3V3 | SCL | SDA | GND | 5V | D8 | GND | 5V | D3 | D4 | 3v3 | 5v | FLASH | RESET

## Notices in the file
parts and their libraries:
SparkFun-PowerSymbols: Licensing: Creative Commons ShareAlike 4.0 International - https://creativecommons.org/licenses/by-sa/4.0
